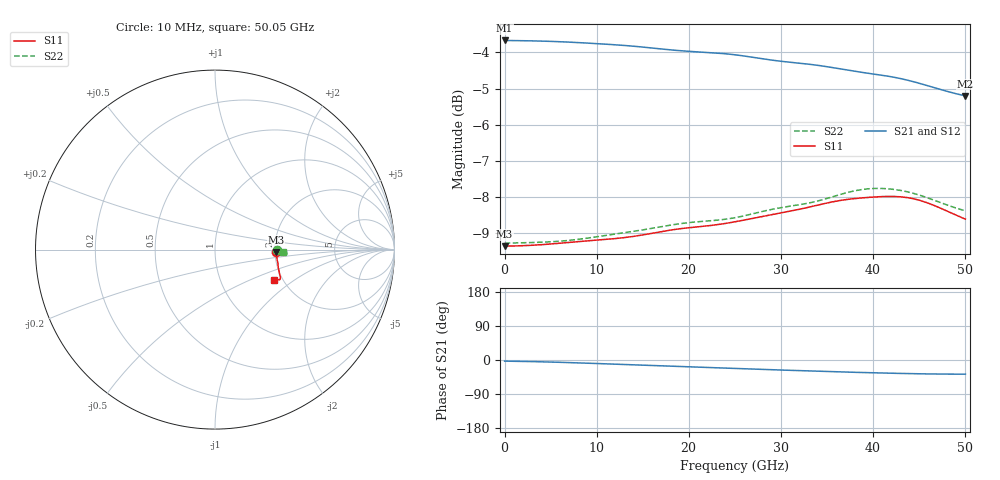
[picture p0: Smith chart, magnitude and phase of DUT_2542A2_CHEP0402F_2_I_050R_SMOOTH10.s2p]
! Touchstone file from project
! Exported from ElectronicsDesktop 2025.1.3
# GHz S MA R 50.000000
! Terminal data exported
! Port[1] = Port1
! Port[2] = Port2
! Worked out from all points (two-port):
!   144 points, 10 MHz to 50.05 GHz, reference 50 ohm
!   highest |S21| = -3.67 dB at 10 MHz (marker M1); lowest = -5.2 dB at 50.05 GHz (marker M2)
!   |S21| within 3 dB of the highest: start of sweep to end of sweep
!   lowest |S11| = -9.4 dB at 10 MHz (marker M3), VSWR 2.03, Z = 101 - j2.89 ohm
!   |S11| at or under -10 dB: nowhere
!   |S22| runs from -9.3 to -7.8 dB; largest |S21 - S12| = 0.0072
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0.01  0.34 -2.1  0.6556 -3.0  0.6553 -2.7  0.3432 -0.5
! Gamma 0 0 0 0
! Port Impedance 50 0 50 0
2.1097  0.3405 -3.1  0.655 -3.8  0.6544 -3.5  0.3437 -1.2
4.2094  0.3417 -4.1  0.6541 -4.9  0.6532 -4.7  0.3444 -1.8
6.3091  0.3435 -5.1  0.6527 -6.3  0.6515 -6.1  0.3457 -2.3
8.4088  0.3453 -6.3  0.6507 -7.9  0.6493 -7.8  0.348 -2.8
10.5085  0.347 -7.5  0.6484 -9.7  0.647 -9.5  0.3511 -3.0
12.95815  0.3493 -8.9  0.6453 -11.8  0.644 -11.6  0.3548 -3.1
16.8076  0.3558 -11.1  0.6384 -15.1  0.6376 -14.9  0.3614 -3.3
19.6072  0.3601 -12.7  0.6337 -17.5  0.6333 -17.3  0.366 -3.6
22.75675  0.3636 -14.9  0.6301 -20.3  0.6301 -20.0  0.369 -4.0
25.2064  0.3678 -16.4  0.6259 -22.4  0.626 -22.1  0.3727 -4.3
28.7059  0.3752 -18.2  0.6165 -25.4  0.6169 -25.1  0.3816 -4.3
33.6052  0.3865 -21.2  0.6065 -29.3  0.6065 -29.0  0.3916 -4.2
36.05485  0.3926 -22.2  0.5999 -31.1  0.5993 -30.8  0.3995 -3.7
38.5045  0.3963 -23.0  0.5929 -32.8  0.5918 -32.5  0.4068 -2.8
40.25425  0.3978 -23.7  0.5886 -33.9  0.5874 -33.5  0.4088 -2.2
42.004  0.3985 -24.4  0.5838 -34.9  0.5827 -34.4  0.4079 -1.9
43.75375  0.397 -25.0  0.5776 -35.8  0.5764 -35.3  0.4044 -1.9
45.15355  0.3933 -25.4  0.5713 -36.4  0.5702 -35.9  0.3998 -2.0
47.6032  0.3826 -26.1  0.5594 -37.2  0.5582 -36.5  0.3897 -2.1
49.003  0.3756 -26.5  0.5532 -37.3  0.5521 -36.6  0.3841 -2.2
50.05285  0.3706 -26.8  0.5493 -37.3  0.5481 -36.6  0.3806 -2.2
